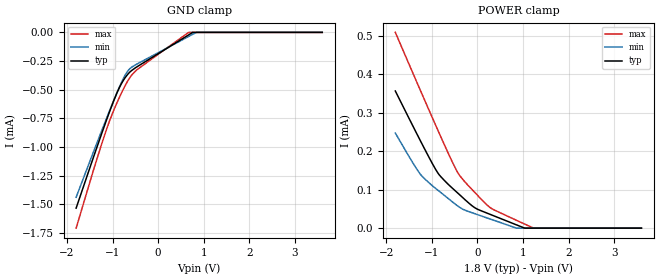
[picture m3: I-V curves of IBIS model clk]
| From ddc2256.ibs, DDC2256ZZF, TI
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|   clk Model
[Model]   clk
Model_type   Input
Vinl = 0.54
Vinh = 1.26
|   typ   min   max
|   (nom PVT)   (fast PVT)   (slow PVT)
C_comp   2.833e-13   2.633e-13   3.126e-13
| Where nom  PVT is Nominal Process, 1.8V, 27C
|   Fast PVT is Strong Process,  1.9V, 0C
|   Slow PVT is Weak Process,   1.7V, 85C
[Voltage Range]   1.8   1.7   1.9
|Junction Temperature
[Temperature Range]   27   85   0
[Power Clamp Reference]   1.8   1.7   1.9
[GND Clamp Reference]   0   0   0
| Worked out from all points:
|   GND clamp passes 1 mA (typ) near -1.34 V on its own axis
[GND Clamp]
|   Voltage   I(typ)   I(min)   I(max)
-1.8V     -1.532mA   -1.438mA   -1.707mA
-1.224V   -865uA     -841.4uA   -953.1uA
-1.067V   -691.8uA   -683.3uA   -771.9uA
-910.9mV  -534.3uA   -532uA     -619.8uA
-786.6mV  -433.7uA   -420.7uA   -513.1uA
-675mV    -369uA     -341.2uA   -428.9uA
-585mV    -333.5uA   -304.6uA   -374.4uA
-468.1mV  -300.9uA   -276.6uA   -326.9uA
668.1mV   -22.1uA    -35.92uA   -34.63nA
757.8mV   -111nA     -16.94uA   0A
838.4mV   0A         0A         0A
3.6V      0A         0A         0A
[POWER Clamp]
|   Voltage   I(typ)   I(min)   I(max)
-1.8V     356.2uA    247uA      508.4uA
-1.246V   226uA      139.3uA    356.6uA
-980.6mV  166.2uA    109.5uA    284.9uA
-840.6mV  139uA      96.11uA    247.5uA
-538.4mV  102.7uA    67.28uA    169uA
-401.6mV  88.04uA    55.08uA    138.8uA
-80.5mV   54.96uA    38.49uA    95.79uA
253.9mV   37.01uA    24.79uA    55.84uA
858.8mV   8.478uA    0A         20.29uA
1.039V    0A         0A         10.55uA
1.229V    0A         0A         0A
3.6V      0A         0A         0A
